| TEXAS INSTRUMENTS INCORPORATED
| Standard Linear and Logic Group
| IBIS Model of SN74CBTD3384C
| 10-Bit FET Bus Switch with -2V Undershoot-Protection and Level
| Shifting
| This file contains package information for the following:
|  SOIC 24-pin (DW) package as [Component] CBTD3384C_DW
|  SSOP 24-pin (DB) package as [Component] CBTD3384C_DB
|  SSOP 24-pin (DBQ) package as [Component] CBTD3384C_DBQ
|  TSSOP 24-pin (PW) package as [Component] CBTD3384C_PW
|  TVSOP 24-pin (DGV) package as [Component] CBTD3384C_DGV
| This device can be powered at the following Vccs:
|  5 volt Vcc
|  4 volt Vcc
| This file provides unique models under the [Model Selector] for each Vcc.
| For operation at a specific Vcc, select the appropriate model after each
| [Model Selector] keyword.
[IBIS Ver]   3.2
[Comment char]  |_char
[File Name]   sn74cbtd3384c.ibs
[File Rev]   1.1 | d_die
[Date]   July 9, 2003
[Source]   Data created from TI-SPICE simulations at TI-SLL.
[Notes]   The following is an IBIS list for the CBTD3384C.
   Please contact sllibis@ti.com with questions and
   comments concerning SLL IBIS models.
   - Power-clamp data has been deleted since there is no
   power-clamp diode in the device.
   - Non-monotonic data due to FET characteristics.
[Disclaimer] Property of Texas Instruments Incorporated.  Unauthorized
   reproduction and/or distribution is strictly prohibited.
   This product is protected under copyright law.
   Created  2003, (C) Copyright  2003, Texas Instruments
   Incorporated, All Rights Reserved
   UNLESS THERE IS A SIGNED, WRITTEN AGREEMENT TO THE
   CONTRARY, TEXAS INSTRUMENTS (TI) IS PROVIDING THE IBIS
   MODELS  AND WITHOUT ANY WARRANTY, EXPRESSED OR
   IMPLIED.  TI assumes no liability for:
   1) the accuracy of the IBIS models provided to your
   company;
   2) the proper functioning of these IBIS Models in your
   design or for any resulting applications; or
   3) infringement of patents, copyrights or intellectual
   property rights resulting from your use of these IBIS
   models.
   TI provides IBIS Models as a service to our customers.
   You and your company shall not distribute, sell or give
   these models to anyone else without prior written
   permission from TI.
   TI reserves the right to make changes to our products or
   to discontinue any semiconductor product or service
   without notice, and advises our customers to obtain the
   latest version of relevant information to verify, before
   placing orders, that the information being relied on is
   current.
   Please be aware that your receipt and use of the IBIS
   information provided shall serve as acceptance of these
   terms and conditions.  If you do not accept these terms,
   you should return or destroy the IBIS models and any
   other accompanying information immediately.
| Component CBTD3384C_DW 24-pin SOIC
[Component]   CBTD3384C_DW
[Manufacturer]   Texas Instruments, Inc.
[Package]
|   typ   min   max
R_pkg   3.700e-02   3.000e-02   4.700e-02
L_pkg   5.146e-09   3.993e-09   6.885e-09
C_pkg   7.580e-13   5.120e-13   1.067e-12
[Pin]   signal_name   model_name   R_pin   L_pin   C_pin
1   1NOE   CBTD3384C_IN   3.900e-02   6.885e-09   1.067e-12
2   1B1   CBTD3384C_IO   4.200e-02   5.950e-09   9.580e-13
3   1A1   CBTD3384C_IO   4.700e-02   5.317e-09   7.910e-13
4   1A2   CBTD3384C_IO   3.100e-02   4.651e-09   6.110e-13
5   1B2   CBTD3384C_IO   3.000e-02   3.993e-09   5.120e-13
6   1B3   CBTD3384C_IO   3.000e-02   4.083e-09   6.110e-13
7   1A3   CBTD3384C_IO   3.000e-02   4.083e-09   6.110e-13
8   1A4   CBTD3384C_IO   3.000e-02   3.993e-09   5.120e-13
9   1B4   CBTD3384C_IO   3.100e-02   4.652e-09   6.110e-13
10   1B5   CBTD3384C_IO   4.700e-02   5.317e-09   7.910e-13
11   1A5   CBTD3384C_IO   4.200e-02   5.950e-09   9.590e-13
12   GND   GND   3.900e-02   6.885e-09   1.067e-12
13   2NOE   CBTD3384C_IN   3.900e-02   6.885e-09   1.067e-12
14   2A1   CBTD3384C_IO   4.200e-02   5.950e-09   9.590e-13
15   2B1   CBTD3384C_IO   4.700e-02   5.317e-09   7.910e-13
16   2B2   CBTD3384C_IO   3.100e-02   4.652e-09   6.110e-13
17   2A2   CBTD3384C_IO   3.000e-02   3.993e-09   5.120e-13
18   2A3   CBTD3384C_IO   3.000e-02   4.083e-09   6.100e-13
19   2B3   CBTD3384C_IO   3.000e-02   4.083e-09   6.100e-13
20   2B4   CBTD3384C_IO   3.000e-02   3.993e-09   5.120e-13
21   2A4   CBTD3384C_IO   3.100e-02   4.651e-09   6.110e-13
22   2A5   CBTD3384C_IO   4.700e-02   5.317e-09   7.910e-13
23   2B5   CBTD3384C_IO   4.200e-02   5.950e-09   9.580e-13
24   VCC   POWER   3.900e-02   6.885e-09   1.067e-12
| Component CBTD3384C_DB 24-pin SSOP
[Component]   CBTD3384C_DB
[Manufacturer]   Texas Instruments, Inc.
[Package]
|   typ   min   max
R_pkg   4.500e-02   4.000e-02   4.900e-02
L_pkg   3.668e-09   3.226e-09   4.415e-09
C_pkg   4.160e-13   3.490e-13   5.070e-13
[Pin]   signal_name   model_name   R_pin   L_pin   C_pin
1   1NOE   CBTD3384C_IN   4.200e-02   4.299e-09   5.030e-13
2   1B1   CBTD3384C_IO   4.000e-02   3.960e-09   4.990e-13
3   1A1   CBTD3384C_IO   4.200e-02   3.775e-09   4.170e-13
4   1A2   CBTD3384C_IO   4.700e-02   3.487e-09   3.690e-13
5   1B2   CBTD3384C_IO   4.600e-02   3.347e-09   3.520e-13
6   1B3   CBTD3384C_IO   4.900e-02   3.352e-09   3.710e-13
7   1A3   CBTD3384C_IO   4.600e-02   3.226e-09   3.630e-13
8   1A4   CBTD3384C_IO   4.700e-02   3.289e-09   3.490e-13
9   1B4   CBTD3384C_IO   4.700e-02   3.347e-09   3.610e-13
10   1B5   CBTD3384C_IO   4.100e-02   3.576e-09   4.090e-13
11   1A5   CBTD3384C_IO   4.100e-02   3.995e-09   5.030e-13
12   GND   GND   4.500e-02   4.415e-09   5.070e-13
13   2NOE   CBTD3384C_IN   4.300e-02   4.337e-09   5.060e-13
14   2A1   CBTD3384C_IO   4.200e-02   4.003e-09   5.040e-13
15   2B1   CBTD3384C_IO   4.100e-02   3.686e-09   4.100e-13
16   2B2   CBTD3384C_IO   4.800e-02   3.355e-09   3.490e-13
17   2A2   CBTD3384C_IO   4.700e-02   3.301e-09   3.530e-13
18   2A3   CBTD3384C_IO   4.800e-02   3.268e-09   3.660e-13
19   2B3   CBTD3384C_IO   4.800e-02   3.269e-09   3.660e-13
20   2B4   CBTD3384C_IO   4.700e-02   3.314e-09   3.490e-13
21   2A4   CBTD3384C_IO   4.800e-02   3.399e-09   3.550e-13
22   2A5   CBTD3384C_IO   4.100e-02   3.688e-09   4.120e-13
23   2B5   CBTD3384C_IO   4.200e-02   4.003e-09   5.040e-13
24   VCC   POWER   4.300e-02   4.347e-09   5.050e-13
| Component CBTD3384C_DBQ 24-pin SSOP
[Component]   CBTD3384C_DBQ
[Manufacturer]   Texas Instruments, Inc.
[Package]
|   typ   min   max
R_pkg   4.400e-02   3.100e-02   6.600e-02
L_pkg   3.074e-09   2.348e-09   4.044e-09
C_pkg   3.220e-13   2.340e-13   4.460e-13
[Pin]   signal_name   model_name   R_pin   L_pin   C_pin
1   1NOE   CBTD3384C_IN   6.500e-02   4.044e-09   4.290e-13
2   1B1   CBTD3384C_IO   6.600e-02   3.824e-09   4.460e-13
3   1A1   CBTD3384C_IO   3.100e-02   3.011e-09   3.210e-13
4   1A2   CBTD3384C_IO   3.200e-02   2.699e-09   2.590e-13
5   1B2   CBTD3384C_IO   3.500e-02   2.519e-09   2.450e-13
6   1B3   CBTD3384C_IO   3.500e-02   2.348e-09   2.340e-13
7   1A3   CBTD3384C_IO   3.500e-02   2.348e-09   2.340e-13
8   1A4   CBTD3384C_IO   3.500e-02   2.518e-09   2.450e-13
9   1B4   CBTD3384C_IO   3.200e-02   2.699e-09   2.590e-13
10   1B5   CBTD3384C_IO   3.100e-02   3.011e-09   3.210e-13
11   1A5   CBTD3384C_IO   6.600e-02   3.824e-09   4.460e-13
12   GND   GND   6.500e-02   4.044e-09   4.290e-13
13   2NOE   CBTD3384C_IN   6.500e-02   4.044e-09   4.290e-13
14   2A1   CBTD3384C_IO   6.600e-02   3.824e-09   4.460e-13
15   2B1   CBTD3384C_IO   3.100e-02   3.011e-09   3.210e-13
16   2B2   CBTD3384C_IO   3.200e-02   2.699e-09   2.590e-13
17   2A2   CBTD3384C_IO   3.500e-02   2.518e-09   2.450e-13
18   2A3   CBTD3384C_IO   3.500e-02   2.348e-09   2.340e-13
19   2B3   CBTD3384C_IO   3.500e-02   2.348e-09   2.340e-13
20   2B4   CBTD3384C_IO   3.500e-02   2.518e-09   2.450e-13
21   2A4   CBTD3384C_IO   3.200e-02   2.699e-09   2.590e-13
22   2A5   CBTD3384C_IO   3.100e-02   3.011e-09   3.210e-13
23   2B5   CBTD3384C_IO   6.600e-02   3.824e-09   4.460e-13
24   VCC   POWER   6.500e-02   4.044e-09   4.290e-13
| Component CBTD3384C_PW 24-pin TSSOP
[Component]   CBTD3384C_PW
[Manufacturer]   Texas Instruments, Inc.
[Package]
|   typ   min   max
R_pkg   3.900e-02   3.000e-02   4.600e-02
L_pkg   2.685e-09   2.367e-09   3.177e-09
C_pkg   3.200e-13   2.520e-13   4.340e-13
[Pin]   signal_name   model_name   R_pin   L_pin   C_pin
1   1NOE   CBTD3384C_IN   3.700e-02   3.153e-09   4.340e-13
2   1B1   CBTD3384C_IO   3.400e-02   2.629e-09   3.410e-13
3   1A1   CBTD3384C_IO   3.200e-02   2.860e-09   3.470e-13
4   1A2   CBTD3384C_IO   4.200e-02   2.741e-09   2.900e-13
5   1B2   CBTD3384C_IO   4.600e-02   2.600e-09   2.620e-13
6   1B3   CBTD3384C_IO   4.300e-02   2.414e-09   2.660e-13
7   1A3   CBTD3384C_IO   4.200e-02   2.367e-09   2.620e-13
8   1A4   CBTD3384C_IO   4.400e-02   2.461e-09   2.520e-13
9   1B4   CBTD3384C_IO   4.200e-02   2.543e-09   2.740e-13
10   1B5   CBTD3384C_IO   3.000e-02   2.616e-09   3.320e-13
11   1A5   CBTD3384C_IO   3.700e-02   2.670e-09   3.460e-13
12   GND   GND   3.900e-02   3.177e-09   4.330e-13
13   2NOE   CBTD3384C_IN   3.700e-02   3.111e-09   4.310e-13
14   2A1   CBTD3384C_IO   3.700e-02   2.656e-09   3.450e-13
15   2B1   CBTD3384C_IO   3.100e-02   2.739e-09   3.400e-13
16   2B2   CBTD3384C_IO   4.200e-02   2.649e-09   2.820e-13
17   2A2   CBTD3384C_IO   4.600e-02   2.532e-09   2.570e-13
18   2A3   CBTD3384C_IO   4.400e-02   2.425e-09   2.660e-13
19   2B3   CBTD3384C_IO   4.400e-02   2.425e-09   2.660e-13
20   2B4   CBTD3384C_IO   4.600e-02   2.532e-09   2.570e-13
21   2A4   CBTD3384C_IO   4.200e-02   2.648e-09   2.820e-13
22   2A5   CBTD3384C_IO   3.100e-02   2.738e-09   3.390e-13
23   2B5   CBTD3384C_IO   3.600e-02   2.653e-09   3.440e-13
24   VCC   POWER   3.700e-02   3.110e-09   4.310e-13
| Component CBTD3384C_DGV 24-pin TVSOP
[Component]   CBTD3384C_DGV
[Manufacturer]   Texas Instruments, Inc.
[Package]
|   typ   min   max
R_pkg   4.300e-02   3.900e-02   4.700e-02
L_pkg   2.601e-09   2.312e-09   3.626e-09
C_pkg   3.580e-13   2.770e-13   5.950e-13
[Pin]   signal_name   model_name   R_pin   L_pin   C_pin
1   1NOE   CBTD3384C_IN   4.300e-02   3.625e-09   5.950e-13
2   1B1   CBTD3384C_IO   4.000e-02   2.656e-09   4.020e-13
3   1A1   CBTD3384C_IO   3.900e-02   2.338e-09   3.080e-13
4   1A2   CBTD3384C_IO   4.600e-02   2.354e-09   2.770e-13
5   1B2   CBTD3384C_IO   4.500e-02   2.312e-09   2.850e-13
6   1B3   CBTD3384C_IO   4.700e-02   2.318e-09   2.820e-13
7   1A3   CBTD3384C_IO   4.700e-02   2.318e-09   2.820e-13
8   1A4   CBTD3384C_IO   4.500e-02   2.312e-09   2.850e-13
9   1B4   CBTD3384C_IO   4.600e-02   2.353e-09   2.780e-13
10   1B5   CBTD3384C_IO   3.900e-02   2.338e-09   3.080e-13
11   1A5   CBTD3384C_IO   4.100e-02   2.660e-09   4.020e-13
12   GND   GND   4.300e-02   3.625e-09   5.950e-13
13   2NOE   CBTD3384C_IN   4.400e-02   3.626e-09   5.940e-13
14   2A1   CBTD3384C_IO   4.000e-02   2.658e-09   4.020e-13
15   2B1   CBTD3384C_IO   3.900e-02   2.343e-09   3.110e-13
16   2B2   CBTD3384C_IO   4.600e-02   2.353e-09   2.780e-13
17   2A2   CBTD3384C_IO   4.500e-02   2.312e-09   2.850e-13
18   2A3   CBTD3384C_IO   4.700e-02   2.319e-09   2.820e-13
19   2B3   CBTD3384C_IO   4.700e-02   2.319e-09   2.820e-13
20   2B4   CBTD3384C_IO   4.500e-02   2.312e-09   2.850e-13
21   2A4   CBTD3384C_IO   4.600e-02   2.353e-09   2.780e-13
22   2A5   CBTD3384C_IO   3.900e-02   2.337e-09   3.080e-13
23   2B5   CBTD3384C_IO   4.000e-02   2.658e-09   4.020e-13
24   VCC   POWER   4.400e-02   3.626e-09   5.950e-13
[Series Switch Groups]
| Function Group States
On  1 /   | 1A1-1A5->1B1-1B5 1noe low
On  2 /   | 2A1-2A5->2B1-2B5 2noe low
On  1 2 /   | 1noe low, 2noe low, enable both
Off 1 2  /   | 1noe high, 2noe high, disable both
[Series Pin Mapping]   pin_2   model_name   function_table_group
3   2   CBTD3384C_IO_50_S   1
| 3   2   CBTD3384C_IO_40_S   1
4   5   CBTD3384C_IO_50_S   1
| 4   5   CBTD3384C_IO_40_S   1
7   6   CBTD3384C_IO_50_S   1
| 7   6   CBTD3384C_IO_40_S   1
8   9   CBTD3384C_IO_50_S   1
| 8   9   CBTD3384C_IO_40_S   1
11   10   CBTD3384C_IO_50_S   1
| 11   10   CBTD3384C_IO_40_S   1
14   15   CBTD3384C_IO_50_S   2
| 14   15   CBTD3384C_IO_40_S   2
17   16   CBTD3384C_IO_50_S   2
| 17   16   CBTD3384C_IO_40_S   2
18   19   CBTD3384C_IO_50_S   2
| 18   19   CBTD3384C_IO_40_S   2
21   20   CBTD3384C_IO_50_S   2
| 21   20   CBTD3384C_IO_40_S   2
22   23   CBTD3384C_IO_50_S   2
| 22   23   CBTD3384C_IO_40_S   2
| Model CBTD3384C_IN
[Model Selector]   CBTD3384C_IN
CBTD3384C_IN_50   5 volt Vcc
CBTD3384C_IN_40   4 volt Vcc
| Model CBTD3384C_IO
[Model Selector]   CBTD3384C_IO
CBTD3384C_IO_50   5 volt Vcc
CBTD3384C_IO_40   4 volt Vcc
| Model CBTD3384C_IO_S
[Model Selector]   CBTD3384C_IO_S
CBTD3384C_IO_50_S   5 volt Vcc_S
CBTD3384C_IO_40_S   4 volt Vcc_S
[Model]   CBTD3384C_IO_50_S
Model_type  Series_switch
| variable   typ   min   max
C_comp   0   0   0
[Temperature Range]   40   100   -40
| Ambient temperature   25   85   -40
[Voltage range]   5   4.5   5.5
[On]
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[Off]
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[Model]   CBTD3384C_IO_40_S
Model_type  Series_switch
| variable   typ   min   max
C_comp   0   0   0
[Temperature Range]   40   100   -40
| Ambient temperature   25   85   -40
[Voltage range]   4   4   4
[On]
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[Off]
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| Models and submodels in the file (6): CBTD3384C_IN_50 (Input), CBTD3384C_IN_40 (Input), CBTD3384C_IO_50_S (Series_switch), CBTD3384C_IO_50 (Terminator), CBTD3384C_IO_40_S (Series_switch), CBTD3384C_IO_40 (Terminator)
